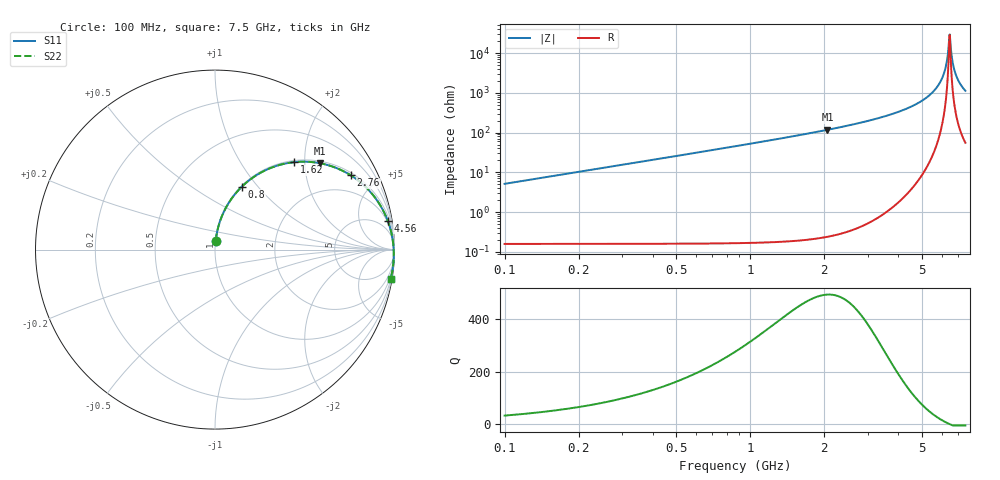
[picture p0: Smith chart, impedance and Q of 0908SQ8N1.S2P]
! Coilcraft 0908SQ-8N1 Air Core Inductor
! 07 March 2008
# MHZ S MA R 50
!Freq  MagS11  AngS11  MagS21  AngS21  MagS12  AngS12  MagS22  AngS22
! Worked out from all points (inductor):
!   371 points, 100 MHz to 7.5 GHz, reference 50 ohm
!   read as one part in series: L = 8.14 nH near 120 MHz
!   highest Q = 493 at 2.06 GHz (marker M1), where L = 9.06 nH
!   self-resonance near 6.46 GHz
!   S11 on the Smith chart (normalised r, x): 100 MHz: 1.00, +0.10; 800 MHz: 1.01, +0.83; 1.62 GHz: 1.03, +1.78; 2.76 GHz: 1.11, +3.59; 4.56 GHz: 2, +12; 7.5 GHz: 1, -12
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100  0.05052 85.3  0.9972 -3.0  0.9972 -3.0  0.05052 85.3
200  0.1007 83.2  0.9934 -5.9  0.9934 -5.9  0.1007 83.2
340  0.1699 79.5  0.9839 -10.0  0.9839 -10.0  0.1699 79.5
800  0.3799 67.0  0.9235 -22.8  0.9235 -22.8  0.38 67.0
1340  0.5778 53.8  0.8147 -36.1  0.8147 -36.1  0.5779 53.8
1620  0.6581 47.8  0.7514 -42.1  0.7514 -42.1  0.6582 47.8
2060  0.7572 39.5  0.6516 -50.4  0.6516 -50.4  0.7573 39.5
2580  0.8405 31.2  0.54 -58.7  0.54 -58.7  0.8405 31.2
2760  0.8626 28.7  0.5037 -61.2  0.5037 -61.2  0.8627 28.7
3800  0.9458 16.5  0.3205 -73.3  0.3205 -73.3  0.9458 16.5
4560  0.9756 9.5  0.2113 -80.0  0.2113 -80.0  0.9756 9.5
5040  0.9864 5.7  0.1508 -83.5  0.1508 -83.5  0.9864 5.7
5860  0.9954 -0.0  0.05984 -87.4  0.05984 -87.4  0.9955 -0.0
6100  0.9964 -1.6  0.03573 -86.8  0.03573 -86.8  0.9964 -1.6
6280  0.9967 -2.7  0.0184 -82.9  0.0184 -82.9  0.9967 -2.7
6360  0.9967 -3.2  0.01101 -76.3  0.01101 -76.3  0.9968 -3.2
6460  0.9967 -3.8  0.003497 -23.4  0.003497 -23.4  0.9967 -3.8
6480  0.9967 -3.9  0.00338 7.7  0.00338 7.7  0.9967 -3.9
6600  0.9965 -4.6  0.01215 69.0  0.01215 69.0  0.9965 -4.6
6780  0.996 -5.6  0.02798 77.0  0.02798 77.0  0.9961 -5.6
7080  0.9947 -7.3  0.05368 78.5  0.05368 78.5  0.9947 -7.3
7500  0.9918 -9.6  0.08779 77.6  0.08779 77.6  0.9919 -9.6
